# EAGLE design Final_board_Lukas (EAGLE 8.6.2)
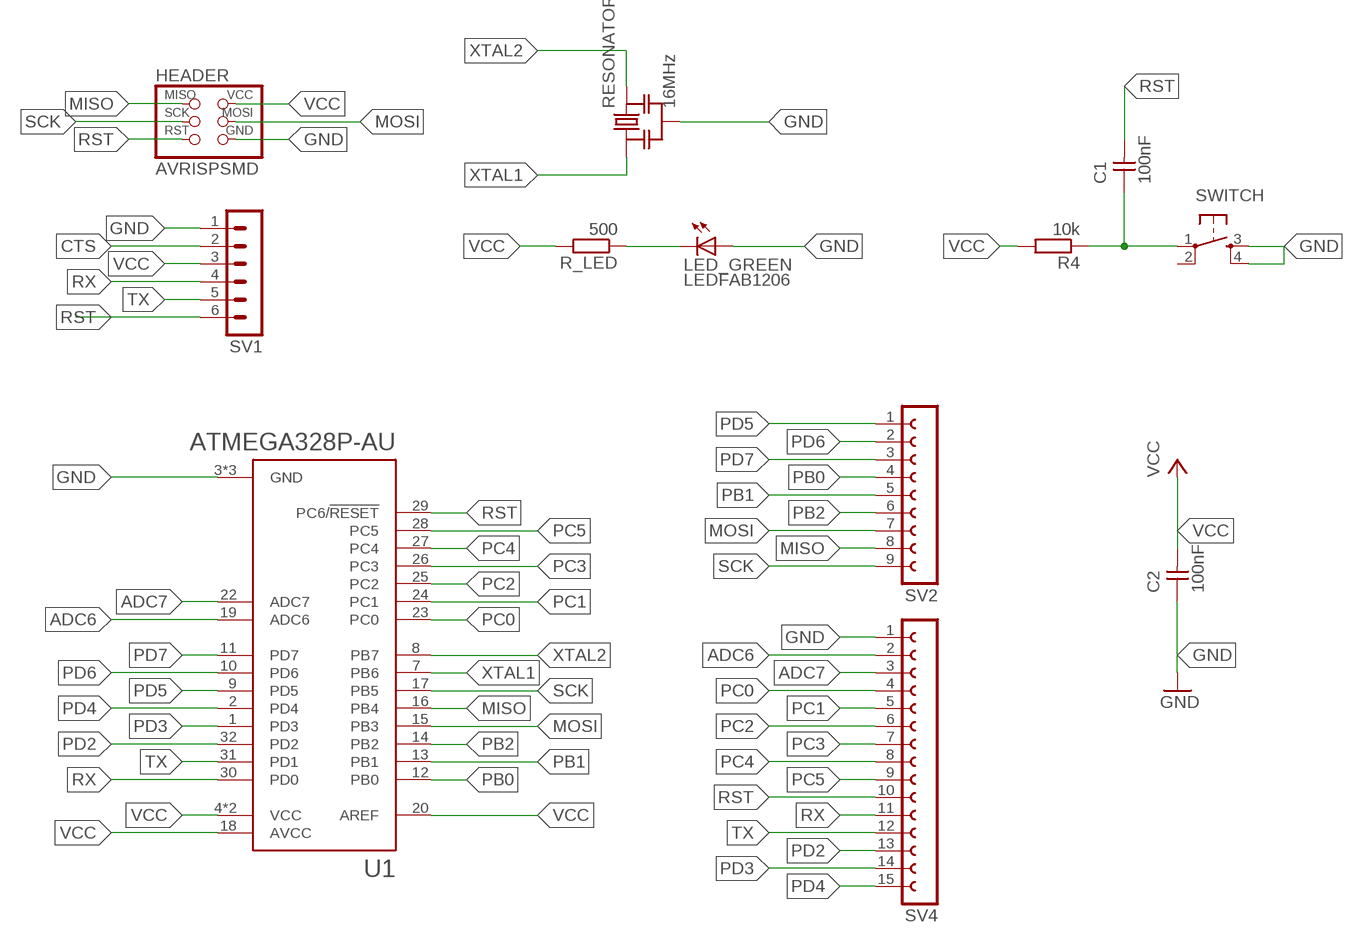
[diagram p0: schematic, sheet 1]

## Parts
C1  100nF  CAP-UNPOLARIZEDFAB  [C1206FAB]
C2  100nF  CAP-UNPOLARIZEDFAB  [C1206FAB]
HEADER  AVRISPSMD  [2X03SMD]
LED_GREEN  LEDFAB1206  [LED1206FAB]
R4  10k  R-EU_R1206  [R1206]
R_LED  500  R-EU_R1206  [R1206]
RESONATOR  16MHz  RESONATOR-MURATACSTCR_G  [RESONATOR_MURATA3]
SV1  MA06-1  [MA06-1]
SV2  FE09-1  [FE09]
SV4  FE15-1  [FE15]
SWITCH  6MM_SWITCH6MM_SWITCH  [6MM_SWITCH]
U1  ATMEGA328P-AU  [QFP80P900X900X120-32N]

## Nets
ADC6: SV4.2 U1.19(ADC6)
ADC7: SV4.3 U1.22(ADC7)
CTS: SV1.2
GND: C2.1 HEADER.6(GND) LED_GREEN.1(A) RESONATOR.2 SV1.1 SV4.1 SWITCH.3(S) SWITCH.4(S1) U1.3(GND) U1.5(GND) U1.21(GND)
MISO: HEADER.1(MISO) SV2.8 U1.16(PB4)
MOSI: HEADER.4(MOSI) SV2.7 U1.15(PB3)
N$21: LED_GREEN.2(C) R_LED.1
PB0: SV2.4 U1.12(PB0)
PB1: SV2.5 U1.13(PB1)
PB2: SV2.6 U1.14(PB2)
PC0: SV4.4 U1.23(PC0)
PC1: SV4.5 U1.24(PC1)
PC2: SV4.6 U1.25(PC2)
PC3: SV4.7 U1.26(PC3)
PC4: SV4.8 U1.27(PC4)
PC5: SV4.9 U1.28(PC5)
PD2: SV4.13 U1.32(PD2)
PD3: SV4.14 U1.1(PD3)
PD4: SV4.15 U1.2(PD4)
PD5: SV2.1 U1.9(PD5)
PD6: SV2.2 U1.10(PD6)
PD7: SV2.3 U1.11(PD7)
RST: C1.1 C1.2 HEADER.5(RST) R4.1 SV1.6 SV4.10 SWITCH.1(P) U1.29(PC6/!RESET)
RX: SV1.4 SV4.11 U1.30(PD0)
SCK: HEADER.3(SCK) SV2.9 U1.17(PB5)
TX: SV1.5 SV4.12 U1.31(PD1)
VCC: C2.2 HEADER.2(VCC) R4.2 R_LED.2 SV1.3 U1.4(VCC) U1.6(VCC) U1.18(AVCC) U1.20(AREF)
XTAL1: RESONATOR.1 U1.7(PB6)
XTAL2: RESONATOR.3 U1.8(PB7)
Unconnected: SWITCH.2(P1)

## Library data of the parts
C1 C2 = fab:CAP-UNPOLARIZED
HEADER = fab:AVRISP
LED_GREEN = fab:LED: LED
R4 R_LED = resistor:R-EU_: RESISTOR, European symbol
RESONATOR = m-pad-2.1:RESONATOR-MURATA: Murata ceramic Resonator "ceralock" CSTCE series with built in load capacitance +- 0.5% tolerance 12.51MHz to 19.99MHz 16MHz murata part#: CSTCE16M0V53-R0 16MHz digikey part#: 490-1198-1-ND $1.33 each
SV1 = con-lstb:MA06-1: PIN HEADER; OC_FARNELL: unknown; OC_NEWARK: unknown
SV2 = con-lsta:FE09-1: FEMALE HEADER; OC_FARNELL: unknown; OC_NEWARK: unknown
SV4 = con-lsta:FE15-1: FEMALE HEADER; OC_FARNELL: unknown; OC_NEWARK: unknown
SWITCH = fab:6MM_SWITCH: OMRON SWITCH
U1 = ATMEGA328P-AU:ATMEGA328P-AU: ATmega Series 20 MHz 32 KB Flash 2 KB SRAM 8-Bit Microcontroller - TQFP-32; AVAILABILITY: Good; DESCRIPTION: ATmega Series 20 MHz 32 KB Flash 2 KB SRAM 8-Bit Microcontroller - TQFP-32; MF: Atmel; MP: ATMEGA328P-AU; PACKAGE: TQFP-32 Atmel; PRICE: 2.38 USD

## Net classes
0 default: clearance 0.205 mm

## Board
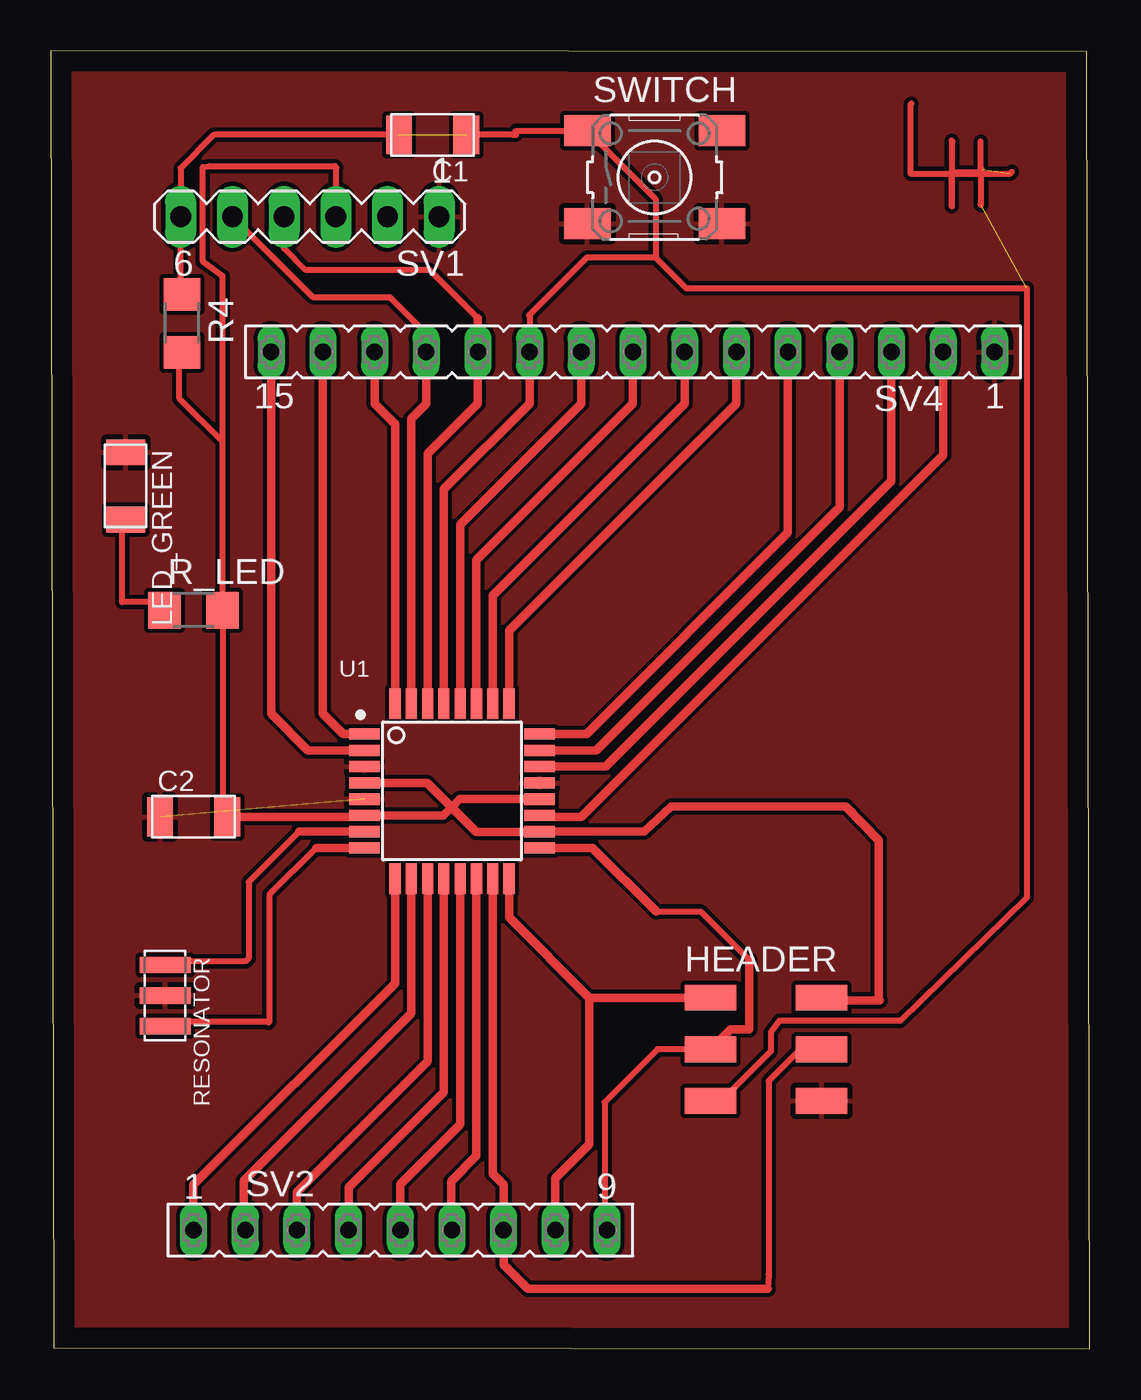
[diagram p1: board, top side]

Size 51.05 x 63.81 mm. Coordinates in mm from the lower left corner, seen from the top.
Outline: 0.14,0.04 51.05,0 50.91,63.77 0,63.81 0.14,0.04
Copper layers (1*16): Top 0.035mm / dielectric 1.5mm / Bottom 0.035mm
Design rules "default *": minimum track width 6mil, minimum drill 0.35mm, track to track 8mil, track to pad 8mil, pad to pad 8mil, via to via 8mil, smd to smd 8mil, copper to edge 40mil, drill to drill 8mil, minimum pad ring 10mil, minimum via ring 8mil, stop-mask expansion 4mil, vias tented up to drill 0mil, thermal gap 10mil

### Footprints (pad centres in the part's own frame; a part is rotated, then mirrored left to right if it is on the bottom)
C1206FAB = smd 1.27 x 1.905: 1 -1.651,0; 2 1.651,0
2X03SMD = smd 2.54 x 1.27: 1 -2.54,2.54; 2 2.92,2.54; 3 -2.54,0; 4 2.92,0; 5 -2.54,-2.54; 6 2.92,-2.54
LED1206FAB = smd 1.27 x 1.905: 1 -1.651,0; 2 1.651,0
R1206 = smd 1.6 x 1.803: 1 -1.422,0; 2 1.422,0
RESONATOR_MURATA3 = smd 0.8 x 2.5: 1 -1.5,0; 2 0,0; 3 1.5,0
MA06-1 = drill 1.016 long: 1 -6.35,0; 2 -3.81,0; 3 -1.27,0; 4 1.27,0; 5 3.81,0; 6 6.35,0
FE09 = drill 0.813 long: 1 -10.16,0; 2 -7.62,0; 3 -5.08,0; 4 -2.54,0; 5 0,0; 6 2.54,0; 7 5.08,0; 8 7.62,0; 9 10.16,0
FE15 = drill 0.813 long: 1 -17.78,0; 2 -15.24,0; 3 -12.7,0; 4 -10.16,0; 5 -7.62,0; 6 -5.08,0; 7 -2.54,0; 8 0,0; 9 2.54,0; 10 5.08,0; 11 7.62,0; 12 10.16,0; 13 12.7,0; 14 15.24,0; 15 17.78,0
6MM_SWITCH = smd 2.286 x 1.524: 1 -3.302,2.286; 2 3.302,2.286; 3 -3.302,-2.286; 4 3.302,-2.286
QFP80P900X900X120-32N = smd 1.5 x 0.55: 1 -4.3,2.8; 2 -4.3,2; 3 -4.3,1.2; 4 -4.3,0.4; 5 -4.3,-0.4; 6 -4.3,-1.2; 7 -4.3,-2; 8 -4.3,-2.8; 17 4.3,-2.8; 18 4.3,-2; 19 4.3,-1.2; 20 4.3,-0.4; 21 4.3,0.4; 22 4.3,1.2; 23 4.3,2; 24 4.3,2.8 | smd 0.55 x 1.5: 9 -2.8,-4.3; 10 -2,-4.3; 11 -1.2,-4.3; 12 -0.4,-4.3; 13 0.4,-4.3; 14 1.2,-4.3; 15 2,-4.3; 16 2.8,-4.3; 25 2.8,4.3; 26 2,4.3; 27 1.2,4.3; 28 0.4,4.3; 29 -0.4,4.3; 30 -1.2,4.3; 31 -2,4.3; 32 -2.8,4.3

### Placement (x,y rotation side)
C1  18.76,59.67 180 top
C2  7.02,26.15 0 top
HEADER  34.96,14.72 0 top
LED_GREEN  3.68,42.42 270 top
R4  6.45,50.41 270 top
R_LED  7.02,36.31 0 top
RESONATOR  5.61,17.36 270 top
SV1  12.73,55.65 180 top
SV2  17.18,5.83 0 top
SV4  28.61,49.01 180 top
SWITCH  29.67,57.59 0 top
U1  19.72,27.42 0 top

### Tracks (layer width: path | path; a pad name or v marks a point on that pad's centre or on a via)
ADC6
  Top 0.406: U1.19 24.09,26.15 26.07,26.15 43.85,43.93 SV4.2
ADC7
  Top 0.406: U1.22 27.27,28.62 41.31,42.66 SV4.3
GND  (1 unrouted)
  pour Top: -46.32,84.57 -46.32,-51.32 -45.05,-52.59 70.52,-52.59 76.87,-46.24 76.87,85.84 66.71,96 -34.89,96
MISO
  Top 0.406: U1.16 22.52,21.2 26.46,17.26 | 26.46,17.26 HEADER.1 | 26.46,17.26 26.46,10.05 24.8,8.38 SV2.8
MOSI
  Top 0.305: HEADER.4 36.84,14.72 35.28,13.16 35.28,3.64 35.24,2.94
  Top 0.406: HEADER.4 37.89,14.7 | 35.24,2.94 23.43,2.94 22.26,4.11 SV2.7 22.26,8.04 21.72,8.59 U1.15
N$21
  Top 0.305: R_LED.1 5.2,36.7 3.51,36.7 3.51,40.6 LED_GREEN.2
  Top 0.406: R_LED.1 5.75,36.46
PB0
  Top 0.406: U1.12 19.32,12.6 14.65,7.94 14.65,5.84 SV2.4
PB1
  Top 0.406: U1.13 20.12,11.02 17.18,8.08 SV2.5
PB2
  Top 0.406: U1.14 20.92,9.47 19.67,8.22 19.67,5.88 SV2.6
PC0
  Top 0.406: U1.23 26.8,29.42 38.77,41.39 SV4.4
PC1
  Top 0.406: U1.24 26.33,30.22 36.23,40.12 SV4.5
PC2
  Top 0.406: U1.25 22.52,35.3 33.69,46.47 SV4.6
PC3
  Top 0.406: U1.26 21.72,37.04 31.15,46.47 SV4.7
PC4
  Top 0.406: U1.27 20.92,38.78 28.61,46.47 SV4.8
PC5
  Top 0.406: U1.28 20.12,40.52 26.07,46.47 SV4.9
PD2
  Top 0.406: U1.32 16.92,45.46 15.91,46.47 SV4.13
PD3
  Top 0.406: U1.1 14.38,30.22 13.37,31.23 SV4.14
PD4
  Top 0.406: U1.2 12.64,29.42 10.83,31.23 SV4.15
PD5
  Top 0.406: U1.9 16.92,17.96 7,8.04 7,5.84 SV2.1
PD6
  Top 0.406: U1.10 17.72,16.48 9.49,8.26 9.49,5.89 SV2.2
PD7
  Top 0.406: U1.11 18.52,14.11 12.1,7.69 SV2.3
RST  (3 unrouted)
  Top 0.305: 6.41,55.62 SV1.6 | SV1.6 6.38,58.04 8.01,59.67 C1.2 | 22.86,59.67 22.68,59.67 | 29.72,53.64 29.72,56.52 SWITCH.1 22.88,59.87 22.68,59.67 | 29.72,53.64 26.34,53.64 23.49,50.79 23.53,50.76 SV4.10 | 29.72,53.64 31.23,52.13 47.96,52.13 47.96,22.2 41.75,16.12 35.81,16.12 35.38,15.56 35.38,14.62 32.94,12.18 HEADER.5 | R4.1 6.38,51.9 SV1.6 | 42.3,61.22 42.26,61.18 42.26,57.78 47.15,57.78 47.23,57.86 | 45.68,57.86 45.66,57.88 45.7,57.92 | 45.7,57.92 45.7,59.35 | 45.7,57.92 45.7,56.25 45.72,56.23 45.72,57.98 | 45.72,57.98 45.74,58 | 45.72,57.98 45.56,57.82 44.31,57.82 44.31,59.35 44.27,59.39 44.27,57.84 | 44.27,57.84 44.27,56.19 44.29,56.17 44.29,57.82 44.27,57.84 | 22.68,59.67 C1.1
  Top 0.406: U1.29 19.32,42.26 23.53,46.47 SV4.10
RX
  Top 0.305: 20.99,50.66 18.59,53.06 12.5,53.06 11.46,54.1 SV1.4
  Top 0.406: U1.30 18.52,44 20.99,46.47 SV4.11 20.99,50.66
SCK
  Top 0.305: 29.74,21.49 31.93,21.49 34.31,19.1 | HEADER.3 29.82,14.72 27.22,12.12 27.22,5.94 SV2.9
  Top 0.406: U1.17 26.61,24.62 29.74,21.49 | HEADER.3 32.43,14.7 33.42,15.69 34.31,15.69 34.31,19.1
TX
  Top 0.305: SV4.12 18.45,49.9 16.64,51.7 12.87,51.7 SV1.5
  Top 0.406: SV4.12 18.45,46.47 17.72,45.74 U1.31
VCC
  Top 0.305: 8.44,44.6 R_LED.2 8.44,26.38 C2.2 | 8.44,44.6 6.32,46.71 6.31,46.71 6.31,48.86 R4.2 | 8.44,44.6 8.44,52.74 7.46,53.45 7.46,58.09 7.79,58.14 13.95,58.14 14.04,58.06 14,58.02 SV1.3
  Top 0.406: U1.4 18.49,27.82 19.69,26.61 | 19.69,26.61 20.91,25.4 24,25.4 U1.18 29.17,25.42 30.49,26.67 39.06,26.67 40.68,24.99 40.68,17.18 40.73,17.13 38.01,17.13 HEADER.2 | 19.69,26.61 19.3,26.22 U1.6 15.35,26.15 C2.2 | U1.20 20.1,27.02 19.69,26.61
XTAL1
  Top 0.305: 12.2,25.42 9.72,22.94 9.72,19.2 9.57,19.05 5.8,19.05 RESONATOR.1
  Top 0.406: U1.7 12.2,25.42
XTAL2
  Top 0.305: 13.03,24.62 10.74,22.32 10.74,16.07 | 10.74,16.07 10.69,16.03 | 10.74,16.07 5.82,16.07 RESONATOR.3
  Top 0.406: U1.8 13.03,24.62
